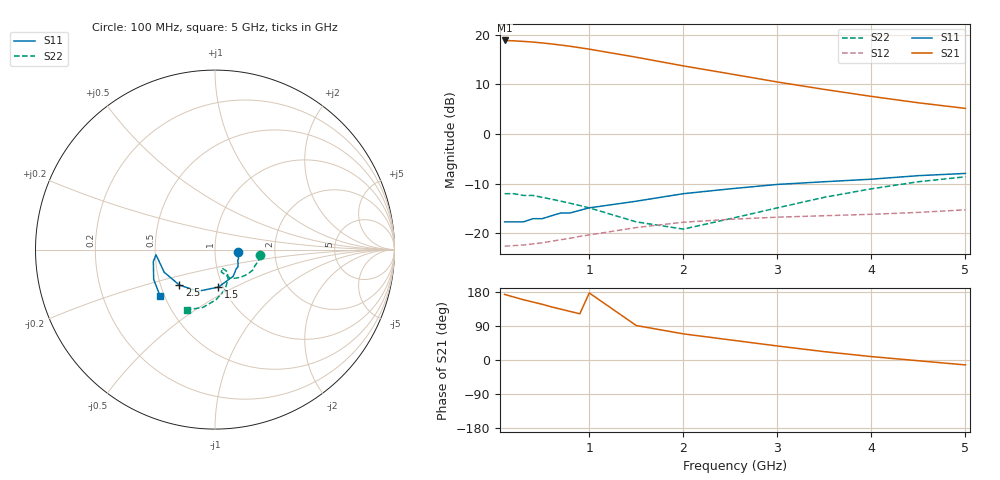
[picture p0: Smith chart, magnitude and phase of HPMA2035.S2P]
! HPMA-2035
! Typical  S-Parameters, Z  = 50, T  = 25 C, I  = 25mA
# ghz s ma r 50
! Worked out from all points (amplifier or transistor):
!   18 points, 100 MHz to 5 GHz, reference 50 ohm
!   highest |S21| = 18.8 dB at 100 MHz (marker M1)
!   |S21| within 3 dB of that: start of sweep to 1.383 GHz
!   unconditionally stable (mu >= 1): start of sweep to end of sweep
!   at 400 MHz: K = 1.06, MAG = 18.8 dB, |S12| = -22.2 dB
!   at 1 GHz: K = 1.00, MAG = 18.5 dB, |S12| = -20.4 dB
!   at 5 GHz: K = 1.35, MAG = 6.7 dB, |S12| = -15.3 dB
!   S11 on the Smith chart (normalised r, x): 100 MHz: 1.30, -0.03; 1.5 GHz: 0.95, -0.42; 2.5 GHz: 0.63, -0.27; 5 GHz: 0.47, -0.29
0.1  0.13 -5.0  8.75 173.0  0.074 3.0  0.25 -7.0
0.2  0.13 -10.0  8.67 166.0  0.075 6.0  0.25 -14.0
0.3  0.13 -15.0  8.56 159.0  0.076 9.0  0.24 -22.0
0.4  0.14 -20.0  8.43 153.0  0.078 12.0  0.24 -28.0
0.5  0.14 -25.0  8.26 147.0  0.08 14.0  0.23 -35.0
0.6  0.15 -31.0  8.07 140.0  0.083 16.0  0.22 -41.0
0.7  0.16 -37.0  7.86 134.0  0.086 18.0  0.21 -47.0
0.8  0.16 -43.0  7.64 128.0  0.089 20.0  0.2 -52.0
0.9  0.17 -50.0  7.39 122.0  0.093 21.0  0.19 -58.0
1  0.18 -56.0  7.15 177.0  0.096 22.0  0.18 -62.0
1.5  0.21 -85.0  5.93 91.0  0.114 23.0  0.13 -74.0
2  0.25 -112.0  4.85 69.0  0.129 21.0  0.11 -69.0
2.5  0.28 -135.0  4.03 53.0  0.138 20.0  0.14 -61.0
3  0.31 -156.0  3.34 37.0  0.145 17.0  0.18 -66.0
3.5  0.33 -175.0  2.81 22.0  0.15 16.0  0.23 -76.0
4  0.35 -169.0  2.39 9.0  0.155 16.0  0.28 -89.0
4.5  0.38 -154.0  2.06 -2.0  0.162 16.0  0.33 -102.0
5  0.4 -140.0  1.81 -13.0  0.172 16.0  0.37 -115.0
